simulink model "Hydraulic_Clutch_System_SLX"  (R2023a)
settings: Solver=ode23s  StartTime=0.0  StopTime=10.0  MaxStep=0.001  RelTol=1e-3
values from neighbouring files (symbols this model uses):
  A_p = 1    [Hydraulic_Clutch_System_EQN.m]    (also in Hydraulic_Clutch_System_SLX_m.m)
  b_7 = 2*N/(m/sec)    (= 2)    [Hydraulic_Clutch_System_EQN.m]    (also in Hydraulic_Clutch_System_SLX_m.m; Car_Dumper_EQN.m; Car_Dumper_SLX_m.m; Electrical_DC_Motor_EQN.m = 0.1)
  C_3 = 0.001*m^3/Pa    (= 0.001)    [Hydraulic_Clutch_System_EQN.m]    (also in Hydraulic_Clutch_System_SLX_m.m; BIG_EC_Simscape_EQN.m; BIG_EC_Simscape_SLX_m.m; Electric_Circuit_03_EQN.m)
  F_8_0 = 0*N    (= 0)    [Hydraulic_Clutch_System_SLX_m.m]    (also in Car_Dumper_SLX_m.m)
  K_8 = 1000*N/m    (= 1000)    [Hydraulic_Clutch_System_EQN.m]    (also in Hydraulic_Clutch_System_SLX_m.m; Car_Dumper_EQN.m; Car_Dumper_SLX_m.m; Rotational_Inertias_and_Dumper_EQN.m = 10)
  M_6 = 0.5*kg    (= 0.5)    [Hydraulic_Clutch_System_EQN.m]    (also in Hydraulic_Clutch_System_SLX_m.m)
  P_1_0 = 10*Pa    (= 10)    [Hydraulic_Clutch_System_SLX_m.m]    (also in Hydraulic_Circuit_01_SLX_m.m; Hydraulic_Circuit_02_SLX_m.m; Hydraulic_Circuit_03_SLX_m.m)
  P_3_0 = 0*Pa    (= 0)    [Hydraulic_Clutch_System_SLX_m.m]
  R_2 = 10000*Pa/(m^3/sec)    (= 10000)    [Hydraulic_Clutch_System_EQN.m]    (also in Hydraulic_Clutch_System_SLX_m.m; BIG_EC_Simscape_EQN.m = 100; BIG_EC_Simscape_SLX_m.m = 100; Electric_Circuit_07_EQN.m = 100)
  Ts = Tfin/Nr_Ts_Points    (= 0.060003)    [Hydraulic_Clutch_System_SLX_m.m]    (also in BIG_EC_Simscape_SLX_m.m = 0.0003; Car_Dumper_SLX_m.m = 0.0022779; Electric_Circuit_01_SLX_m.m = 0.005; Electric_Circuit_02_SLX_m.m = 0.000480145)
  v_6_0 = 0*m/sec    (= 0)    [Hydraulic_Clutch_System_SLX_m.m]
  v_9_0 = 0*m/sec    (= 0)    [Hydraulic_Clutch_System_SLX_m.m]    (also in Car_Dumper_SLX_m.m)

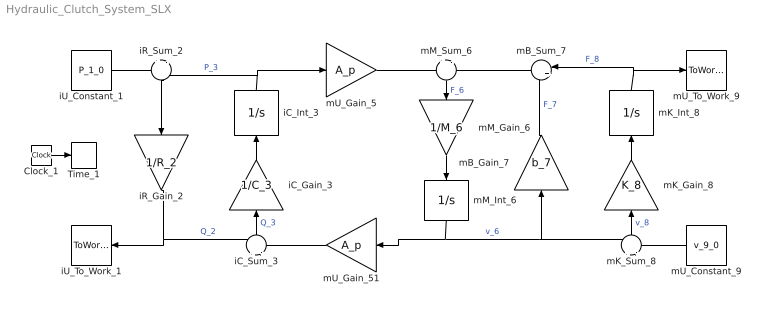
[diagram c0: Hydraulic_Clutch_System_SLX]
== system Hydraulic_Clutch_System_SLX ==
  Clock_1 : Clock
  Time_1 : ToWorkspace  VariableName=t  SaveFormat=Timeseries  SampleTime=Ts
  iC_Gain_3 : Gain  Gain=1/C_3  Multiplication=Matrix(K*u)
  iC_Int_3 : Integrator  InitialCondition=P_3_0
  iC_Sum_3 : Sum  Inputs=+|-
  iR_Gain_2 : Gain  Gain=1/R_2  Multiplication=Matrix(K*u)
  iR_Sum_2 : Sum  Inputs=+|-
  iU_Constant_1 : Constant  Value=P_1_0
  iU_To_Work_1 : ToWorkspace  VariableName=Q_1_0  SaveFormat=Timeseries  SampleTime=Ts
  mB_Gain_7 : Gain  Gain=b_7  Multiplication=Matrix(K*u)
  mB_Sum_7 : Sum  Inputs=|++
  mK_Gain_8 : Gain  Gain=K_8  Multiplication=Matrix(K*u)
  mK_Int_8 : Integrator  InitialCondition=F_8_0
  mK_Sum_8 : Sum  Inputs=+|-
  mM_Gain_6 : Gain  Gain=1/M_6  Multiplication=Matrix(K*u)
  mM_Int_6 : Integrator  InitialCondition=v_6_0
  mM_Sum_6 : Sum  Inputs=+|-
  mU_Constant_9 : Constant  Value=v_9_0
  mU_Gain_5 : Gain  Gain=A_p  Multiplication=Matrix(K*u)
  mU_Gain_51 : Gain  Gain=A_p  Multiplication=Matrix(K*u)
  mU_To_Work_9 : ToWorkspace  VariableName=F_9_0  SaveFormat=Timeseries  SampleTime=Ts
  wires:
  iU_Constant_1/1 -> iR_Sum_2/1
  iC_Int_3/1 -> iR_Sum_2/2, mU_Gain_5/1  "P_3"
  iR_Gain_2/1 -> iU_To_Work_1/1, iC_Sum_3/1  "Q_2"
  iR_Sum_2/1 -> iR_Gain_2/1
  mU_Gain_51/1 -> iC_Sum_3/2
  iC_Sum_3/1 -> iC_Gain_3/1  "Q_3"
  iC_Gain_3/1 -> iC_Int_3/1
  mU_Gain_5/1 -> mM_Sum_6/1
  mM_Int_6/1 -> mU_Gain_51/1, mB_Gain_7/1, mK_Sum_8/1  "v_6"
  mB_Sum_7/1 -> mM_Sum_6/2
  mM_Sum_6/1 -> mM_Gain_6/1  "F_6"
  mM_Gain_6/1 -> mM_Int_6/1
  mK_Int_8/1 -> mB_Sum_7/1, mU_To_Work_9/1  "F_8"
  mB_Gain_7/1 -> mB_Sum_7/2  "F_7"
  mU_Constant_9/1 -> mK_Sum_8/2
  mK_Sum_8/1 -> mK_Gain_8/1  "v_8"
  mK_Gain_8/1 -> mK_Int_8/1
  Clock_1/1 -> Time_1/1
